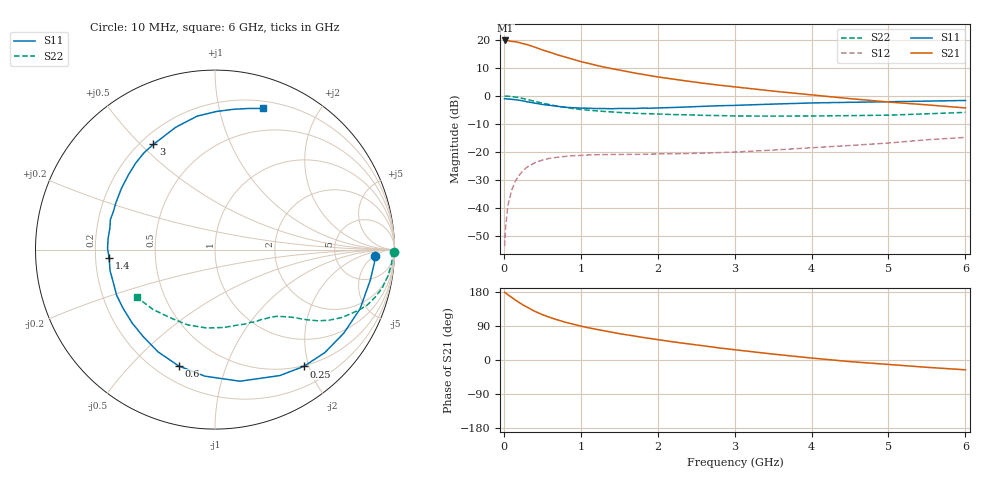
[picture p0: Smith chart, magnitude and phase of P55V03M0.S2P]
! SIEMENS Small Signal Semiconductors
! BFP183
! Si NPN RF Bipolar Junction Transistor in SOT143
! VCE = 5 V  IC = 3 mA
! Common Emitter S-Parameters:  March  1996
# GHz  S  MA  R  50
!  f  S11  S21  S12  S22
! GHz  MAG  ANG  MAG  ANG  MAG  ANG  MAG  ANG
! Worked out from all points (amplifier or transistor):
!   36 points, 10 MHz to 6 GHz, reference 50 ohm
!   highest |S21| = 19.8 dB at 20 MHz (marker M1)
!   |S21| within 3 dB of that: start of sweep to 463.2 MHz
!   unconditionally stable (mu >= 1): 1.887 GHz to 5.725 GHz
!   at 250 MHz: K = 0.15, MSG = 22.6 dB, |S12| = -26.6 dB
!   at 1.4 GHz: K = 0.77, MSG = 15.3 dB, |S12| = -20.9 dB
!   at 6 GHz: K = 0.95, MSG = 5.3 dB, |S12| = -14.8 dB
!   lowest NFmin = 1.10 dB at 450 MHz
!   S11 on the Smith chart (normalised r, x): 10 MHz: 16, -5; 250 MHz: 0.49, -1.92; 600 MHz: 0.29, -0.69; 1.4 GHz: 0.26, -0.04; 3 GHz: 0.25, +0.55; 6 GHz: 0.27, +1.36
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0.01  0.8902 -2.2  9.631 178.7  0.0021 91.0  0.9983 -0.9
0.02  0.8914 -4.6  9.756 177.5  0.0041 87.1  0.987 -1.7
0.05  0.8818 -11.1  9.71 172.6  0.0107 87.0  0.9879 -4.4
0.15  0.8552 -33.0  9.282 158.3  0.0304 71.6  0.9557 -13.0
0.2  0.8388 -43.2  8.941 151.6  0.0388 66.4  0.9297 -16.7
0.25  0.8171 -52.8  8.546 145.3  0.0466 61.8  0.9019 -20.1
0.3  0.7892 -62.8  8.253 139.7  0.0537 57.4  0.8668 -23.0
0.4  0.7463 -79.3  7.44 128.7  0.0642 49.2  0.803 -28.1
0.5  0.7073 -94.6  6.614 119.8  0.0719 43.0  0.7468 -31.8
0.6  0.6789 -107.4  6.01 112.2  0.0775 38.0  0.6986 -34.6
0.7  0.6522 -119.1  5.39 105.7  0.0809 33.7  0.6565 -36.7
0.8  0.6282 -129.7  4.934 99.6  0.0837 30.8  0.624 -38.4
1  0.6076 -147.5  4.102 89.5  0.087 25.9  0.5744 -41.1
1.1  0.6042 -155.2  3.808 85.0  0.0887 24.3  0.5572 -42.3
1.4  0.5916 -175.3  3.075 73.5  0.0905 20.8  0.5198 -45.9
1.8  0.6065 164.0  2.432 59.8  0.0912 19.5  0.4854 -51.0
2.2  0.6227 146.9  1.997 47.9  0.0931 20.0  0.4658 -57.1
3  0.6793 120.3  1.453 27.1  0.1 23.0  0.4399 -72.3
3.5  0.7159 107.8  1.221 15.6  0.1084 24.7  0.4368 -83.2
4.5  0.7702 89.2  0.896 -4.3  0.131 25.4  0.4462 -110.1
5.5  0.8086 76.5  0.694 -19.3  0.1657 23.2  0.4806 -136.2
6  0.8306 71.2  0.612 -25.9  0.1821 19.8  0.5095 -148.6
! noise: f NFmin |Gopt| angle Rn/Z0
0.45  1.1  0.37  35  0.3
0.9  1.15  0.34  85  0.23
1.8  1.9  0.35  160  0.13
